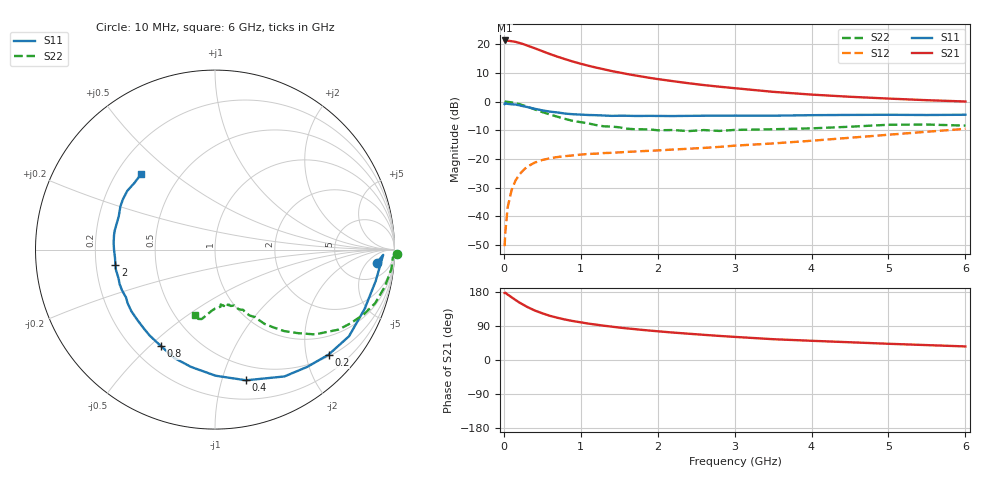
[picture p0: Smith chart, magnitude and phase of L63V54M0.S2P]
!  INFINEON TECHNOLOGIES Small Signal Semiconductors
! BFR380L3 , Si-NPN RF-Transistor in TSLP-3-1
!  Vce=3.5 V,  Ic=4 mA
! Common Emitter S-Parameters:  07. March 2005
#  GHz  S  MA  R  50
! f  S11  S21  S12  S22
! GHz  Mag  Ang  Mag  Ang  Mag  Ang  Mag  Ang
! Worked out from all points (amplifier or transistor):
!   36 points, 10 MHz to 6 GHz, reference 50 ohm
!   highest |S21| = 21.3 dB at 10 MHz (marker M1)
!   |S21| within 3 dB of that: start of sweep to 428.9 MHz
!   unconditionally stable (mu >= 1): 2.639 GHz to 4.653 GHz
!   at 250 MHz: K = 0.14, MSG = 22.1 dB, |S12| = -24.0 dB
!   at 1.4 GHz: K = 0.70, MSG = 14.3 dB, |S12| = -17.9 dB
!   at 6 GHz: K = 0.92, MSG = 4.8 dB, |S12| = -9.5 dB
!   S11 on the Smith chart (normalised r, x): 10 MHz: 12, -10; 200 MHz: 0.54, -2.45; 400 MHz: 0.36, -1.20; 800 MHz: 0.31, -0.54; 2 GHz: 0.28, -0.07; 6 GHz: 0.30, +0.39
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0.01  0.9034 -4.7  11.65 176.8  0.003 84.3  1.013 -1.3
0.02  0.9374 -1.8  11.58 177.4  0.0054 95.1  0.9915 -2.6
0.05  0.9122 -11.1  11.55 172.6  0.0143 84.4  0.9888 -6.3
0.1  0.8966 -21.7  11.3 165.7  0.0283 79.0  0.9682 -12.4
0.15  0.8891 -32.9  11.03 158.6  0.0415 72.5  0.941 -18.5
0.2  0.8619 -42.8  10.57 151.9  0.053 68.4  0.9042 -23.5
0.3  0.8057 -61.3  9.541 140.4  0.0725 59.5  0.8191 -33.0
0.4  0.7485 -76.6  8.535 130.8  0.086 52.9  0.7305 -40.3
0.5  0.7027 -89.7  7.58 123.2  0.0956 48.4  0.656 -45.2
0.6  0.6672 -101.5  6.742 116.5  0.1026 44.8  0.595 -49.7
0.7  0.6449 -110.7  6.054 111.3  0.1079 42.4  0.5418 -53.1
0.8  0.6163 -119.2  5.48 106.6  0.1118 40.8  0.4974 -56.3
0.9  0.6016 -127.2  4.977 102.7  0.1149 39.6  0.4579 -58.3
1.1  0.5832 -138.3  4.216 96.0  0.1219 38.9  0.4156 -62.2
1.5  0.5656 -156.2  3.219 85.6  0.1299 39.6  0.3559 -68.5
2  0.5609 -171.4  2.47 75.8  0.1405 42.6  0.3158 -75.9
2.2  0.5592 -175.7  2.268 72.4  0.1456 44.4  0.3186 -76.4
2.8  0.5683 172.0  1.819 63.6  0.1619 49.7  0.3074 -84.0
3.5  0.5672 161.0  1.479 54.9  0.186 54.1  0.329 -90.0
4.5  0.5847 151.3  1.213 46.8  0.2337 60.1  0.3641 -96.8
5.5  0.5828 140.6  1.057 39.3  0.2973 61.7  0.3975 -103.6
6  0.5889 134.3  1.003 35.8  0.3345 61.1  0.3806 -106.8
